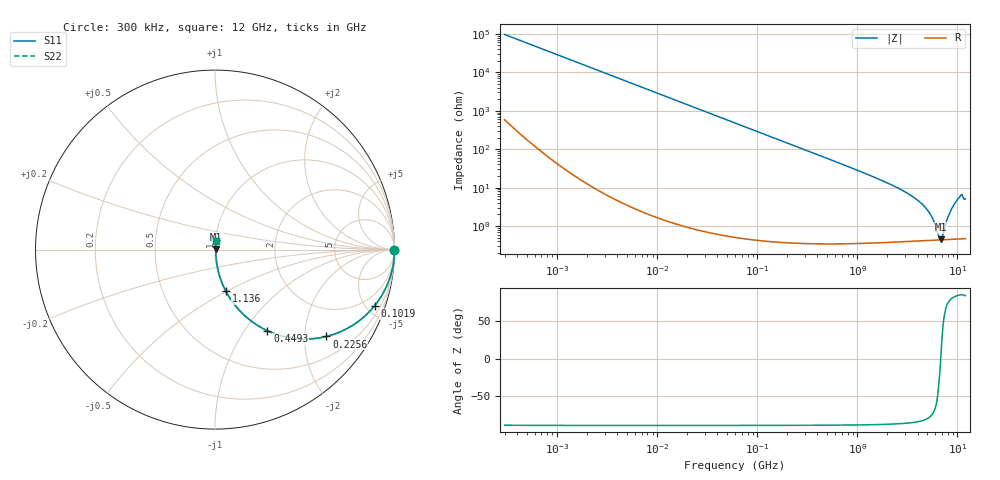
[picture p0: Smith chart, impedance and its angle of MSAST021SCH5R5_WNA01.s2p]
! MSAST021SCH5R5_WNA01  S-PARAMETER MODEL  ( General Type )
! Model Generated by TAIYO YUDEN Corporation (http://www.ty-top.com)
! Version 2.0
! TAIYO YUDEN Control No. 181101
! Copyright(c) 2015 TAIYO YUDEN CO.,LTD. All Rights Reserved.
! Product Description (link to TY-COMPAS)
! https://ds.yuden.co.jp/TYCOMPAS/or/detail?pn=MSAST021SCH5R5CWNA01&u=M
! Products Name : Multilayer Ceramic Capacitors
! Characteristics :
!  Capacitance : 5.5 pF , Rated Voltage : 25V , TCC : CH / C0H
!  Case Size : 0.25 x 0.125 / 0.0098 x 0.0049 [mm/inch] , Thickness : 0.125 / 0.0049 [mm/inch]
!  (Conditions: Temperature = 25 degC , DC Bias Current/Voltage = 0A / 0V)
! External Node Assignments :
!  1  o---| |---o  2
! GND o---------o GND
! Frequency Range : 0.3MHz  -  12000MHz  [ 401 STEP ]
# MHz S RI R 50
! Freq[MHz].  S11 Real  S11 Imag  S21 Real  S21 Imag  S12 Real  S12 Imag  S22 Real  S22 Imag
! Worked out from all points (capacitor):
!   401 points, 300 kHz to 12 GHz, reference 50 ohm
!   read as one part in series: C = 5.5 pF near 316.3 kHz
!   lowest |Z| = 447 mohm at 6.88 GHz (marker M1)
!   series resonance near 6.805 GHz, so ESL is about 99 pH
!   S11 on the Smith chart (normalised r, x): 300 kHz: open; 101.9 MHz: 1.01, -5.68; 225.6 MHz: 1.01, -2.56; 449.3 MHz: 1.01, -1.28; 1.136 GHz: 1.01, -0.50; 12 GHz: 1.01, +0.10
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0.3  1 -0.00104  7.35e-06 0.00104  7.35e-06 0.00104  1 -0.00104
1.769972  1 -0.00612  4.31e-05 0.00612  4.31e-05 0.00612  1 -0.00612
10.44266  0.9987 -0.036  0.00132 0.036  0.00132 0.036  0.9987 -0.036
60  0.9586 -0.1987  0.0414 0.1987  0.0414 0.1987  0.9586 -0.1987
101.9188  0.8892 -0.3131  0.1108 0.3131  0.1108 0.3131  0.8892 -0.3131
225.6362  0.621 -0.4837  0.379 0.4837  0.379 0.4837  0.621 -0.4837
353.9943  0.3997 -0.4877  0.6003 0.4877  0.6003 0.4877  0.3997 -0.4877
449.3064  0.2924 -0.4522  0.7076 0.4522  0.7076 0.4522  0.2924 -0.4522
704.9044  0.1436 -0.3465  0.8564 0.3465  0.8564 0.3465  0.1436 -0.3465
1135.593  0.0607 -0.2317  0.9393 0.2317  0.9393 0.2317  0.0607 -0.2317
2088.533  0.019 -0.1224  0.981 0.1224  0.981 0.1224  0.019 -0.1224
3276.641  0.00844 -0.0666  0.9916 0.0666  0.9916 0.0666  0.00844 -0.0666
4502.883  0.00538 -0.0352  0.9946 0.0352  0.9946 0.0352  0.00538 -0.0352
5420.343  0.00459 -0.0187  0.9954 0.0187  0.9954 0.0187  0.00459 -0.0187
5868.704  0.00442 -0.0118  0.9956 0.0118  0.9956 0.0118  0.00442 -0.0118
6524.734  0.00435 -0.00274  0.9957 0.00274  0.9957 0.00274  0.00435 -0.00274
6879.757  0.00437 0.000845  0.9956 -0.000845  0.9956 -0.000845  0.00437 0.000845
7254.098  0.00443 0.00531  0.9956 -0.00531  0.9956 -0.00531  0.00443 0.00531
8281.503  0.00486 0.0197  0.9951 -0.0197  0.9951 -0.0197  0.00486 0.0197
9454.42  0.00608 0.039  0.9939 -0.039  0.9939 -0.039  0.00608 0.039
10511.28  0.00774 0.0558  0.9923 -0.0558  0.9923 -0.0558  0.00774 0.0558
12000  0.00719 0.05  0.9928 -0.05  0.9928 -0.05  0.00719 0.05
